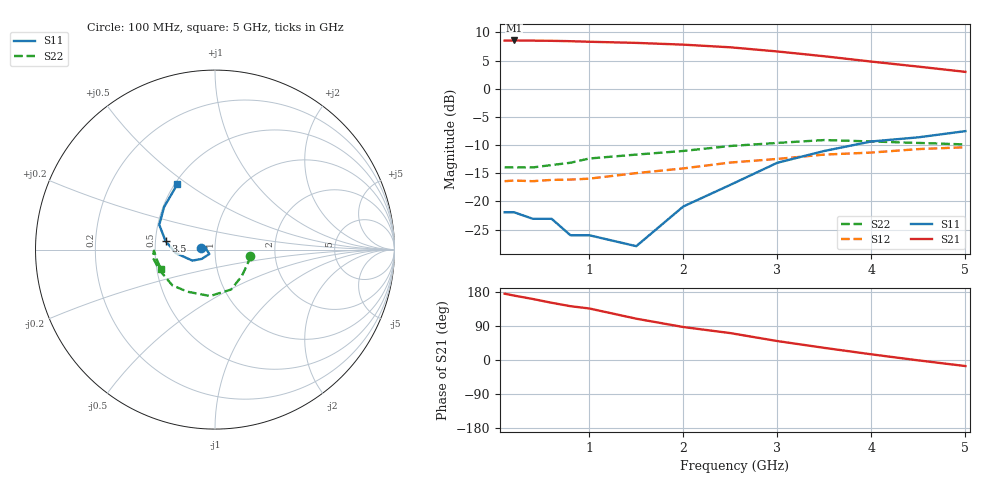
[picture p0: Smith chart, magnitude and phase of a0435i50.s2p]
!  MSA-0435 S AND NOISE PARAMETERS
!  Id=50mA  LAST UPDATED 07-22-92
# ghz s ma r 50
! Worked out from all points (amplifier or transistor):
!   14 points, 100 MHz to 5 GHz, reference 50 ohm
!   highest |S21| = 8.6 dB at 200 MHz (marker M1)
!   |S21| within 3 dB of that: start of sweep to 3.602 GHz
!   unconditionally stable (mu >= 1): start of sweep to 3.332 GHz
!   at 400 MHz: K = 1.37, MAG = 8.8 dB, |S12| = -16.4 dB
!   at 2 GHz: K = 1.16, MAG = 8.5 dB, |S12| = -14.2 dB
!   at 5 GHz: K = 0.95, MSG = 6.7 dB, |S12| = -10.4 dB
!   lowest NFmin = 6.10 dB at 100 MHz
!   S11 on the Smith chart (normalised r, x): 100 MHz: 0.85, +0.01; 3.5 GHz: 0.57, +0.06; 5 GHz: 0.52, +0.46
0.1  0.08 175.0  2.67 175.0  0.151 1.0  0.2 -10.0
0.2  0.08 172.0  2.68 170.0  0.153 2.0  0.2 -16.0
0.4  0.07 171.0  2.67 161.0  0.151 3.0  0.2 -33.0
0.6  0.07 166.0  2.66 151.0  0.155 6.0  0.21 -45.0
0.8  0.05 169.0  2.64 142.0  0.156 8.0  0.22 -57.0
1  0.05 175.0  2.61 136.0  0.159 10.0  0.24 -68.0
1.5  0.04 -142.0  2.55 109.0  0.178 13.0  0.26 -96.0
2  0.09 -145.0  2.46 87.0  0.196 15.0  0.28 -123.0
2.5  0.14 -154.0  2.33 71.0  0.221 18.0  0.31 -140.0
3  0.22 -175.0  2.14 50.0  0.238 14.0  0.33 -160.0
3.5  0.28 170.0  1.94 32.0  0.26 9.0  0.35 -173.0
4  0.34 156.0  1.74 15.0  0.271 4.0  0.34 -179.0
4.5  0.37 140.0  1.57 -1.0  0.291 -2.0  0.33 -171.0
5  0.42 120.0  1.41 -16.0  0.302 -8.0  0.32 -160.0
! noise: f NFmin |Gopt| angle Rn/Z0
0.1  6.1  0.12  -178  0.66
0.5  6.1  0.13  -170  0.65
1  6.4  0.15  -160  0.66
2  7.2  0.21  -140  0.68
